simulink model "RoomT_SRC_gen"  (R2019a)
settings: Solver=ode15s  StartTime=0.0  StopTime=tend  RelTol=1e-3
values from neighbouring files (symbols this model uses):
  ACmax = 4.5    [mainV3.m]    (also in mainV3_SRC.m)
  ACmin = 0    [mainV3.m]    (also in mainV3_SRC.m)
  alphaAC = -abs(a(1))    [StdSRC_3MVs.m]
  alphaEH = abs(a(3))    [StdSRC_3MVs.m]
  alphaHW = abs(a(2))    [StdSRC_3MVs.m]
  EHmax = 4    [mainV3.m]    (also in mainV3_SRC.m)
  EHmin = 0    [mainV3.m]    (also in mainV3_SRC.m)
  HWmax = 3    [mainV3.m]    (also in mainV3_SRC.m)
  HWmin = 0    [mainV3.m]    (also in mainV3_SRC.m)
  Kc_SRC = abs(double(S.Kc))    [StdSRC_3MVs.m]    (also in TuningSRC.m = abs(Kc_SRC))
  KI_SRC = Kc_SRC/tauISRC    [StdSRC_3MVs.m]    (also in TuningSRC.m = Kc_SRC/tauI_SRC)
  m_in0 = 0.4    [mainOL.m]    (also in mainV3.m; mainV3_SRC.m)
  p = [m,Cp, Ufl, Afl, mfl, Cpfl]'    [mainOL.m]    (also in mainV3.m; mainV3_SRC.m)
  par_J = [p_el, p_hw, p_ac, m_in0, kv, kT]'    [mainV3.m]    (also in mainV3_SRC.m)
  Tdes0 = T0    (= 21)    [mainV3.m]    (also in mainV3_SRC.m)
  Tin0 = 21    [mainOL.m]    (also in mainV3.m; mainV3_SRC.m)
  Tin_1 = 0    [mainOL.m]    (also in mainV3.m = 10; mainV3_SRC.m = 10)
  Tin_2 = 0    [mainOL.m]    (also in mainV3.m = -5; mainV3_SRC.m = -5)
  Tin_3 = -8    [mainV3.m]    (also in mainV3_SRC.m)
  Tin_4 = -13    [mainV3.m]    (also in mainV3_SRC.m)
  Tin_5 = +13    (= 13)    [mainV3.m]    (also in mainV3_SRC.m = 0)
  tTin_1 = 190000    [mainOL.m]    (also in mainV3.m = 1800; mainV3_SRC.m = 1800)
  tTin_2 = 2    [mainOL.m]    (also in mainV3.m = 12600; mainV3_SRC.m = 12600)
  tTin_3 = 7*3600    (= 25200)    [mainV3.m]    (also in mainV3_SRC.m)
  tTin_4 = 10*3600    (= 36000)    [mainV3.m]    (also in mainV3_SRC.m)
  tTin_5 = 10012.0*3600    (= 36043200)    [mainV3.m]    (also in mainV3_SRC.m = 20000)
  u0AC = 0    [StdSRC_3MVs.m]
  u0EH = -abs((dv(2))*(alphaEH))    [StdSRC_3MVs.m]
  u0HW = 0    [StdSRC_3MVs.m]
  x0 = [T0; Tfl0]    [mainOL.m]    (also in mainV3.m; mainV3_SRC.m; col_obj.m = 0.5*ones(1,82)'; Simulate1Col.m = x)
undefined symbols (not defined in the file or in its folder): objRoom, Room, SR_block
libraries: simulink x1

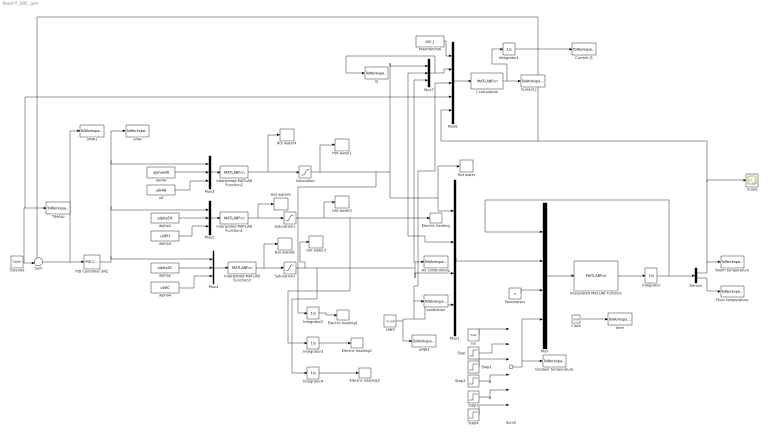
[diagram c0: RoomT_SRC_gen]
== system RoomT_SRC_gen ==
  Air conditioning : ToWorkspace  VariableName=QAC  SampleTime=-1
  Clock : Clock
  Current J : ToWorkspace  VariableName=Jactual  SampleTime=-1
  Current J1 : ToWorkspace  VariableName=Jtot  SampleTime=-1
  Demux : Demux  Outputs=2
  Electric heating : ToWorkspace  VariableName=QH2  SampleTime=-1
  Electric heating1 : ToWorkspace  VariableName=E_HW  SampleTime=-1
  Electric heating2 : ToWorkspace  VariableName=E_EH  SampleTime=-1
  Electric heating3 : ToWorkspace  VariableName=E_AC  SampleTime=-1
  Floor temperature : ToWorkspace  VariableName=Tfl  SampleTime=-1
  HW3 : Constant  Value=m_in0
  Hot water : ToWorkspace  VariableName=QH1  SampleTime=-1
  Hot water1 : ToWorkspace  VariableName=uHW  SampleTime=-1
  Hot water2 : ToWorkspace  VariableName=uEH  SampleTime=-1
  Hot water3 : ToWorkspace  VariableName=uAC  SampleTime=-1
  Hot water4 : ToWorkspace  VariableName=uHW1  SampleTime=-1
  Hot water5 : ToWorkspace  VariableName=uEH1  SampleTime=-1
  Hot water6 : ToWorkspace  VariableName=uAC1  SampleTime=-1
  Integrator : Integrator  InitialCondition=x0'
  Integrator{1..4} (4 alike) : Integrator
  Interpreted MATLAB Function : MATLABFcn  MATLABFcn=Room(u)  OutputDimensions=2  Output1D=off
  Interpreted MATLAB Function1 : MATLABFcn  MATLABFcn=SR_block(u)  OutputDimensions=1
  Interpreted MATLAB Function2 : MATLABFcn  MATLABFcn=SR_block(u)  OutputDimensions=1
  Interpreted MATLAB Function3 : MATLABFcn  MATLABFcn=SR_block(u)  OutputDimensions=1
  J calculation : MATLABFcn  MATLABFcn=objRoom(u)  OutputDimensions=1  Output1D=off
  Mux : Mux
  Mux1 : Mux
  Mux{2..4,7} (4 alike) : Mux  Inputs=3
  Mux6 : Mux  Inputs=5
  Outdoor temperature : ToWorkspace  VariableName=Tin  SampleTime=-1
  PID Controller SRC : simulink/Continuous/PID Controller  Controller=PI  Form=Parallel  TimeDomain=Continuous-time  SampleTime=-1  IntegratorMethod=Forward Euler  FilterMethod=Forward Euler  ControllerParametersSource=internal  P=Kc_SRC  I=KI_SRC  D=0  UseFilter=on  N=100  TunerSelectOption=Transfer Function Based (PID Tuner App)  InitialConditionSource=internal  InitialConditionForIntegrator=0  InitialConditionForFilter=0  DifferentiatorICPrevScaledInput=0  ExternalReset=none  TrackingMode=off  Kt=1  LimitOutput=off  UpperSaturationLimit=HWmax  LowerSaturationLimit=HWmin  LinearizeAsGain=on  AntiWindupMode=clamping  Kb=1  POutMin=[]  POutMax=[]  IOutMin=[]  IOutMax=[]  DOutMin=[]  DOutMax=[]  NOutMin=[]  NOutMax=[]  SumOutMin=[]  SumOutMax=[]  SaturationOutMin=[]  SaturationOutMax=[]  PParamMin=[]  PParamMax=[]  IParamMin=[]  IParamMax=[]  DParamMin=[]  DParamMax=[]  NParamMin=[]  NParamMax=[]  KbParamMin=[]  KbParamMax=[]  KtParamMin=[]  KtParamMax=[]  KbOutMin=[]  KbOutMax=[]  KtOutMin=[]  KtOutMax=[]  IntegratorOutMin=[]  IntegratorOutMax=[]  FilterOutMin=[]  FilterOutMax=[]  SumI1OutMin=[]  SumI1OutMax=[]  SumI2OutMin=[]  SumI2OutMax=[]  SumI3OutMin=[]  SumI3OutMax=[]  SumI4OutMin=[]  SumI4OutMax=[]  SumDOutMin=[]  SumDOutMax=[]  DifferentiatorOutMin=[]  DifferentiatorOutMax=[]  FilterDiffOutCoefMin=[]  FilterDiffOutCoefMax=[]  ReciprocalOutMin=[]  ReciprocalOutMax=[]  SumDenOutMin=[]  SumDenOutMax=[]  SumNumOutMin=[]  SumNumOutMax=[]  DivideOutMin=[]  DivideOutMax=[]  IntegratorContinuousStateAttributes=''  IntegratorStateMustResolveToSignalObject=off  IntegratorRTWStateStorageClass=Auto  FilterContinuousStateAttributes=''  FilterStateMustResolveToSignalObject=off  FilterRTWStateStorageClass=Auto  ParallelPVariant=InternalParameters  IdealPVariant=Disabled  IVariant=InternalParameters  DVariant=Disabled  IntegratorVariant=Continuous  SatVariant=Disabled  AWVariant=Passthrough  PCopyVariant=Disabled  TRVariant=Disabled  FdbkBlocksVariant=Forward  IdealPFdbkVariant=Disabled  SatFdbkVariant=Disabled  DerivativeFilterVariant=Disabled  NVariant=Disabled  NCopyVariant=Disabled_SignalSpec  FilterICVariant=Disabled  IntegratorICVariant=InternalICs  ExternalResetVariant=Disabled  TRSumVariant=Passthrough  SumFdbkVariant=Disabled  SumVariant=Sum_PI
  Parameters : Constant  Value=p
  Parameters6 : Constant  Value=par_J
  Q : ToWorkspace  VariableName=Q  SampleTime=-1
  Room temperature : ToWorkspace  VariableName=T  SampleTime=-1
  Saturation : Saturate  UpperLimit=HWmax  LowerLimit=HWmin
  Saturation1 : Saturate  UpperLimit=EHmax  LowerLimit=EHmin
  Saturation2 : Saturate  UpperLimit=ACmax  LowerLimit=ACmin
  Scope : Scope
  Step : Step  Time=tTin_1  After=Tin_1  SampleTime=0
  Step1 : Step  Time=tTin_2  After=Tin_2  SampleTime=0
  Step2 : Step  Time=tTin_3  After=Tin_3  SampleTime=0
  Step3 : Step  Time=tTin_4  After=Tin_4  SampleTime=0
  Step4 : Step  Time=tTin_5  After=Tin_5  SampleTime=0
  Sum : Sum  Inputs=-+|
  Sum2 : Sum  Inputs=|++++++
  Tdesired : Constant  Value=Tdes0
  Tdessp : ToWorkspace  VariableName=Tdes_sp  SampleTime=-1
  Tin : Constant  Value=Tin0
  alpha : Constant  Value=alphaHW
  alpha1 : Constant  Value=alphaEH
  alpha2 : Constant  Value=alphaAC
  alpha3 : Constant  Value=u0EH
  alpha4 : Constant  Value=u0AC
  time : ToWorkspace  VariableName=t  SampleTime=-1
  u0 : Constant  Value=u0HW
  uHW : ToWorkspace  VariableName=v  SampleTime=-1
  uHW1 : ToWorkspace  VariableName=e  SampleTime=-1
  uHW3 : ToWorkspace  VariableName=u_mv  SampleTime=-1
  ventilation : ToWorkspace  VariableName=m_in  SampleTime=-1
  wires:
  Clock/1 -> time/1
  Interpreted MATLAB Function/1 -> Integrator/1
  Mux/1 -> Interpreted MATLAB Function/1
  Integrator/1 -> Demux/1, Mux/1
  Parameters/1 -> Mux/3
  Sum2/1 -> Mux/4, Outdoor temperature/1
  Step1/1 -> Sum2/3
  Step/1 -> Sum2/2
  Tin/1 -> Sum2/1
  Mux1/1 -> Mux/2
  Demux/1 -> Mux6/5, Sum/1, Scope/1, Room temperature/1
  Demux/2 -> Floor temperature/1
  PID Controller SRC/1 -> Mux4/1, Mux2/1, Mux3/1, uHW/1
  Interpreted MATLAB Function1/1 -> Hot water5/1, Saturation1/1
  Interpreted MATLAB Function3/1 -> Hot water6/1, Saturation2/1
  Step2/1 -> Sum2/4
  Step3/1 -> Sum2/5
  Step4/1 -> Sum2/6
  J calculation/1 -> Integrator1/1, Current J/1
  Mux6/1 -> J calculation/1
  HW3/1 -> Mux6/3, ventilation/1, Mux1/4, uHW3/1
  Parameters6/1 -> Mux6/1
  Mux7/1 -> Q/1, Mux6/2
  Interpreted MATLAB Function2/1 -> Hot water4/1, Saturation/1
  Mux2/1 -> Interpreted MATLAB Function1/1
  Mux3/1 -> Interpreted MATLAB Function2/1
  Mux4/1 -> Interpreted MATLAB Function3/1
  alpha/1 -> Mux3/2
  alpha1/1 -> Mux2/2
  alpha2/1 -> Mux4/2
  u0/1 -> Mux3/3
  alpha3/1 -> Mux2/3
  alpha4/1 -> Mux4/3
  Tdesired/1 -> Mux6/4, Tdessp/1, Sum/2
  Sum/1 -> uHW1/1, PID Controller SRC/1
  Saturation/1 -> Hot water1/1, Integrator2/1, Hot water/1, Mux1/1, Mux7/1
  Saturation1/1 -> Hot water2/1, Integrator3/1, Mux1/2, Mux7/2, Electric heating/1
  Saturation2/1 -> Hot water3/1, Integrator4/1, Mux1/3, Mux7/3, Air conditioning/1
  Integrator1/1 -> Current J1/1
  Integrator4/1 -> Electric heating3/1
  Integrator2/1 -> Electric heating1/1
  Integrator3/1 -> Electric heating2/1
